(* Logix 5000 DataType export AMCI_5034_PTO_AM_Output_Data; software revision 37.00 *)

TYPE AMCI_5034_PTO_AM_Output_Data :
STRUCT
   Command_Word : DINT;
   TargetPosition : DINT;
   TargetVelocity : UDINT;
   Acceleration : DINT;
   Deceleration : DINT;
END_STRUCT
END_TYPE
